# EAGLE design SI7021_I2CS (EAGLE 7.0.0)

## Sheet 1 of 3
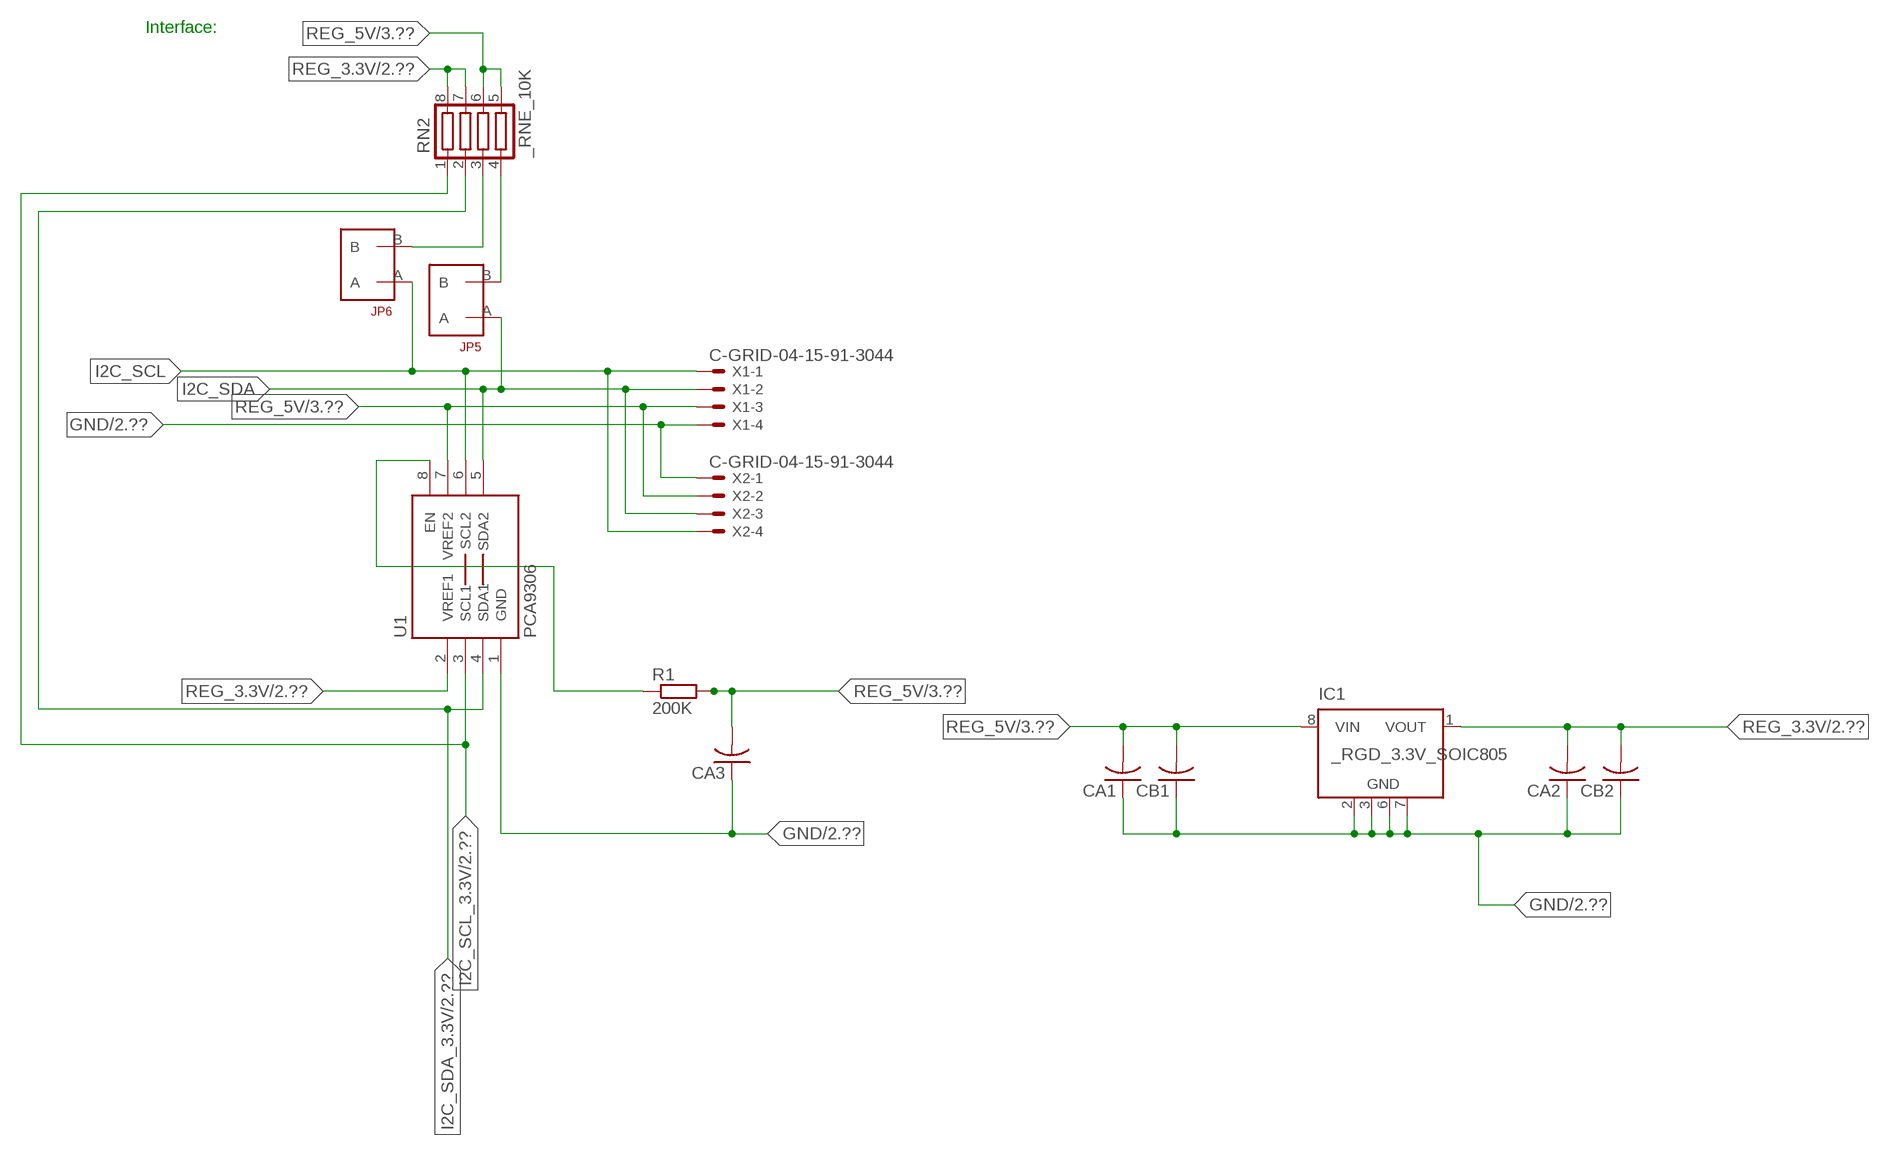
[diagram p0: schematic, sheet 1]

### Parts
CA1  CC1206KRX7R9BB104  [.1UF]
CA2  CC1206KRX7R9BB104  [.1UF]
CA3  CC1206KRX7R9BB104  [.1UF]
CB1  TMK316F106ZL-TC1206K  [TMK316F106ZL-T]
CB2  TMK316F106ZL-TC1206K  [TMK316F106ZL-T]
IC1  _RGD_3.3V_SOIC805  [_RGC_3.3V_SOIC8]
JP5  JUMPER_1X2_2MM  [JUMPER_1X2_2MM]
JP6  JUMPER_1X2_2MM  [JUMPER_1X2_2MM]
R1  200K  RESISTOR_SMT-0603  [R603]
RN2  _RNE_10K  [RNE]
U1  PCA9306  PCA9306_NCD  [PSOP-8]
X1  C-GRID-04-15-91-3044  [15-91-04]
X2  C-GRID-04-15-91-3044  [15-91-04]

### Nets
GND: CA1.1 CA2.1 CA3.1 CB1.1 CB2.1 IC1.2(GND) IC1.3(GND) IC1.6(GND) IC1.7(GND) U1.1(GND) X1.4 X2.1 ; also sheet 2,3
I2C_SCL: JP6.A U1.6(SCL2) X1.1 X2.4
I2C_SCL_3.3V: RN2.1 U1.3(SCL1) ; also sheet 2
I2C_SDA: JP5.A U1.5(SDA2) X1.2 X2.3
I2C_SDA_3.3V: RN2.2 U1.4(SDA1) ; also sheet 2
N$1: JP6.B RN2.3
N$2: JP5.B RN2.4
N$3: R1.1 U1.8(EN)
REG_3.3V: CA2.2 CB2.2 IC1.1(VOUT) RN2.7 RN2.8 U1.2(VREF1) ; also sheet 2
REG_5V: CA1.2 CA3.2 CB1.2 IC1.8(VIN) R1.2 RN2.5 RN2.6 U1.7(VREF2) X1.3 X2.2 ; also sheet 3
Unconnected: IC1.4(NC) IC1.5(NC)

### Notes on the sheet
- Interface:

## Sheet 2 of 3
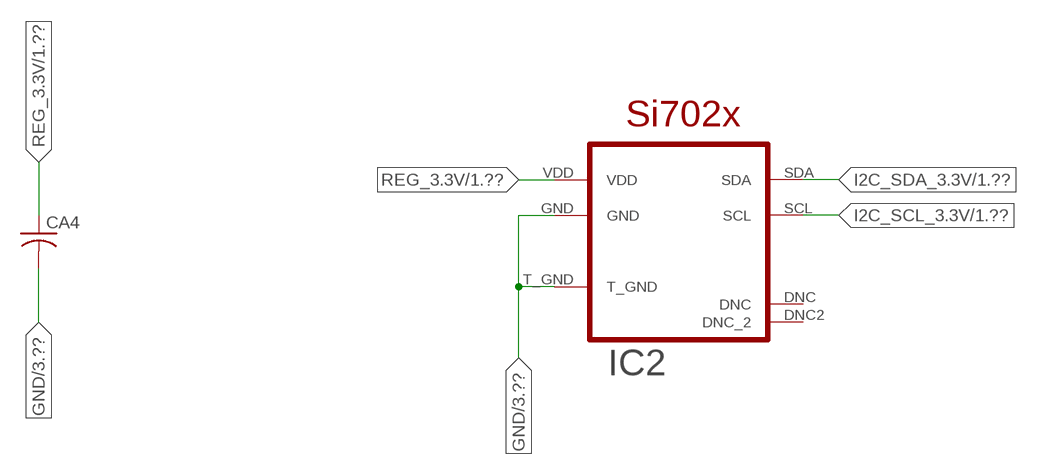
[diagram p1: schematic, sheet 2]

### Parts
CA4  CC1206KRX7R9BB104  [.1UF]
IC2  SI7021  SI702X  [DFN6]

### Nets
GND: CA4.2 IC2.GND IC2.T_GND ; also sheet 1,3
I2C_SCL_3.3V: IC2.SCL ; also sheet 1
I2C_SDA_3.3V: IC2.SDA ; also sheet 1
REG_3.3V: CA4.1 IC2.VDD ; also sheet 1
Unconnected: IC2.DNC IC2.DNC2(DNC_2)

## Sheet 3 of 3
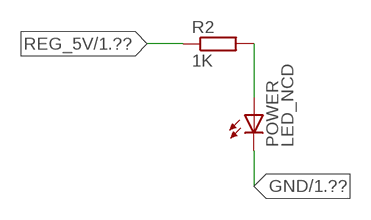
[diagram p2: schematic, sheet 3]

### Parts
POWER  LED_NCD  [CHIPLED_0603]
R2  1K  RESISTOR_SMT-0402  [R402]

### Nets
GND: POWER.C ; also sheet 1,2
N$4: POWER.A R2.2
REG_5V: R2.1 ; also sheet 1

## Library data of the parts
CA1-CA3 = NCD_ULTIMATE_LIBRARY:CC1206KRX7R9BB104: Capacitor CA .1uF 50V SMT C1206K CC1206KRX7R9BB104
CA4 = NCD_ULTIMATE_LIBRARY (1):CC1206KRX7R9BB104: Capacitor CA .1uF 50V SMT C1206K CC1206KRX7R9BB104
CB1 CB2 = NCD_ULTIMATE_LIBRARY:TMK316F106ZL-T: Capacitor CB 10uF SMT 1206 TMK316F106ZL-T
IC1 = NCD_ULTIMATE_LIBRARY:_RGD_3.3V_SOIC8: Regulator Linear 3.3V Chip Positive VOLTAGE REGULATOR Digikey 497-1199-2-ND/L78L33ACD13TR
IC2 = postalecki:SI702X
JP5 JP6 = NCD_ULTIMATE_CONNECTORS:JUMPER_1X2_2MM
POWER = NCD_ULTIMATE_LIBRARY:LED_NCD: LED Digikey 754-1132-2-ND/APT2012SRCPRV
R1 R2 = NCD_ULTIMATE_LIBRARY:RESISTOR_SMT: NCD Resistor
RN2 = NCD_ULTIMATE_LIBRARY:_RNE_10K: Resistor Array RNE SMT 10K x 4 Single Resistor Source: http://www.ctscorp.com/components/Datasheets/CTSChipArrayDs.pdf Digikey 742C083103JPTR-ND/742C083103JP; OC_FARNELL: unknown; OC_NEWARK: unknown
U1 = NCD_ULTIMATE_LIBRARY:PCA9306_NCD: NCD Bidirectional I2C level shifter. NOT compatible with all available part number pinout schemes- DOUBLE CHECK!!!; PROD_ID: IC-10023
X1 X2 = NCD_ULTIMATE_CONNECTORS:C-GRID-04: CONNECTOR 4-Pos I2C wire to board 2.54 mm (0.100") pitch header Digikey WM1342-ND/0015912045; OC_FARNELL: unknown; OC_NEWARK: unknown

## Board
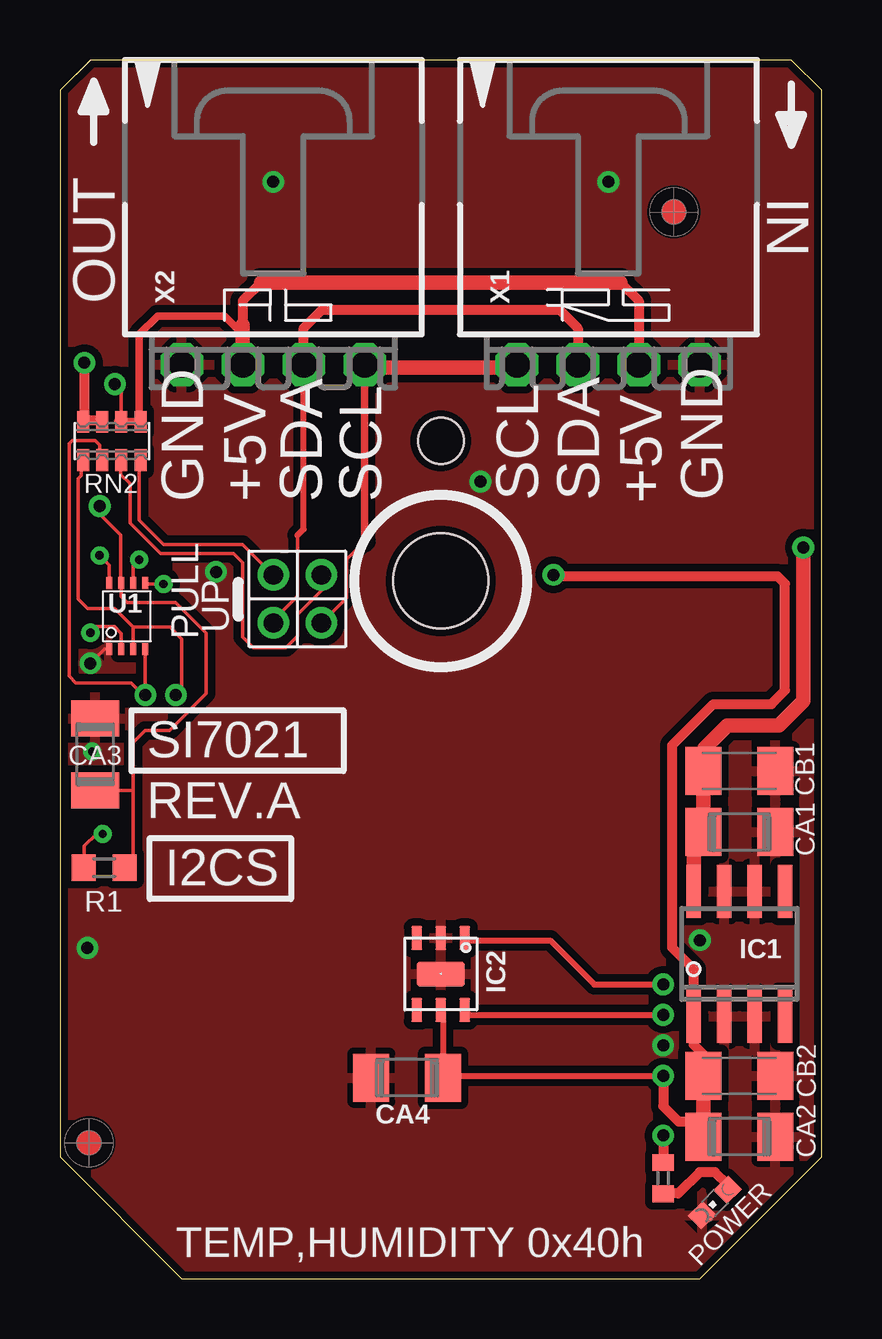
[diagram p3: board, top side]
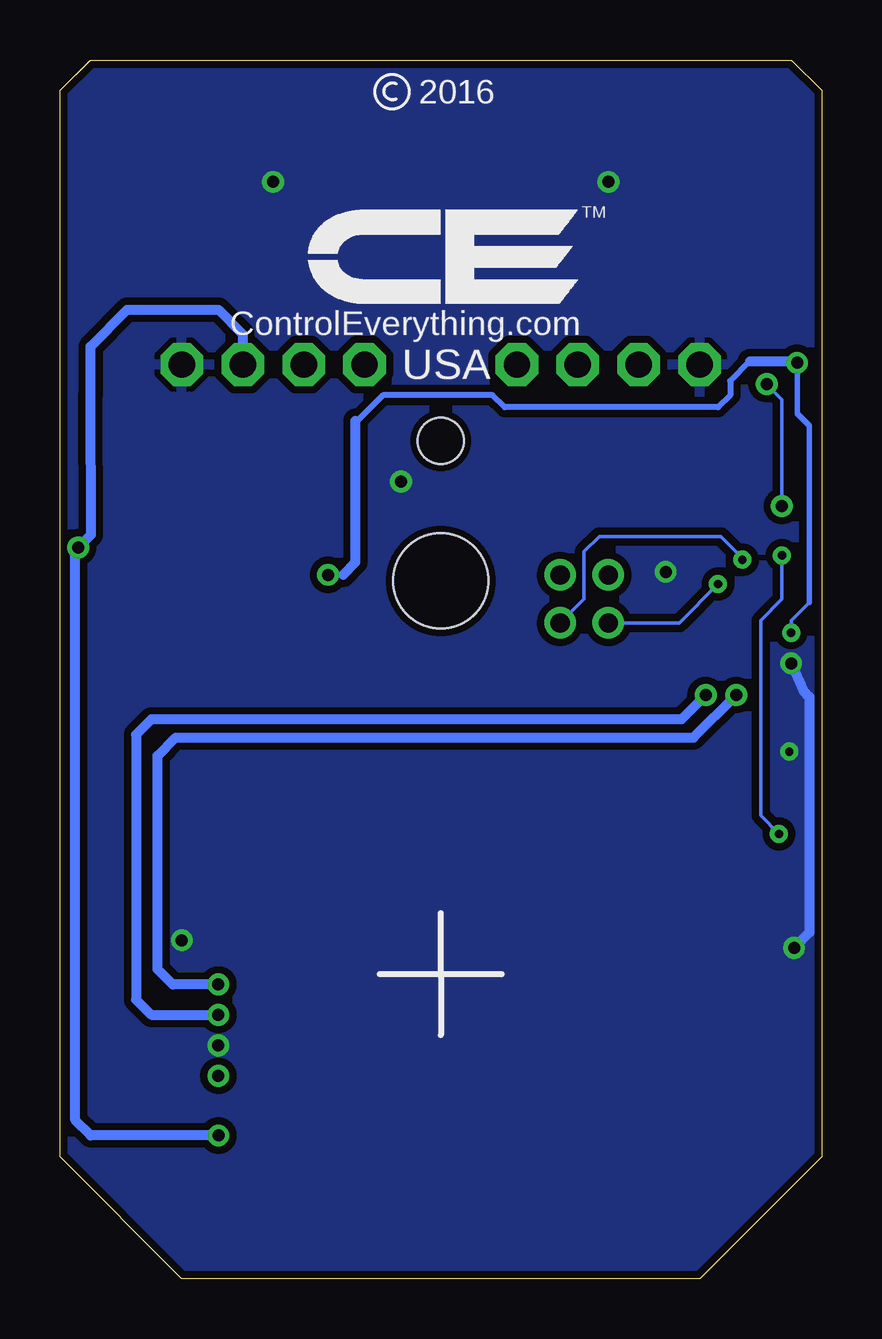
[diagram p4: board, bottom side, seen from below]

Size 31.75 x 50.8 mm. Coordinates in mm from the lower left corner, seen from the top.
Outline: 32 segments
Copper layers (1*16): Top 0.035mm / dielectric 1.5mm / Bottom 0.035mm
Design rules "default": minimum track width 5mil, minimum drill 24mil, track to track 5mil, track to pad 5mil, pad to pad 5mil, via to via 5mil, smd to smd 5mil, copper to edge 10mil, drill to drill 8mil, minimum pad ring 10mil, minimum via ring 8mil, stop-mask expansion 2mil, vias tented up to drill 0mil, thermal gap 10mil
Holes 3.96 mm at 15.88,29.08
Holes 1.91 mm at 15.88,34.93

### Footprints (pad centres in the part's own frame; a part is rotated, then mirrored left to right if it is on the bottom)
.1UF = smd 1.5 x 2: 1 -1.5,0; 2 1.5,0
TMK316F106ZL-T = smd 1.5 x 2: 1 -1.5,0; 2 1.5,0
_RGC_3.3V_SOIC8 = smd 0.6 x 2.2: 1 -1.905,-2.6; 2 -0.635,-2.6; 3 0.635,-2.6; 4 1.905,-2.6; 5 1.905,2.6; 6 0.635,2.6; 7 -0.635,2.6; 8 -1.905,2.6
DFN6 = smd 1 x 0.45: DNC -1.5,-1; DNC2 1.5,-1; GND -1.5,0; SCL 1.5,1; SDA -1.5,1; VDD 1.5,0 | smd 1 x 2: T_GND 0,0
JUMPER_1X2_2MM = drill 0.8: A 0,2; B 0,0
CHIPLED_0603 = smd 0.8 x 0.876: A 0,-0.75; C 0,0.75
R603 = smd 1 x 1.1: 1 -0.85,0; 2 0.85,0
R402 = smd 0.7 x 0.9: 1 -0.65,0; 2 0.65,0
RNE = smd 0.5 x 0.9: 1 -1.2,-0.8; 2 -0.4,-0.8; 3 0.4,-0.8; 4 1.2,-0.8; 5 1.2,0.8; 6 0.4,0.8; 7 -0.4,0.8; 8 -1.2,0.8
PSOP-8 = smd 0.25 x 0.5: 1 -0.73,-1.37; 2 -0.23,-1.37; 3 0.27,-1.37; 4 0.77,-1.37; 5 0.77,1.38; 6 0.27,1.38; 7 -0.23,1.38; 8 -0.73,1.38
15-91-04 = drill 1.1 pad 1.778 octagon: 1 -3.81,-7.62; 2 -1.27,-7.62; 3 1.27,-7.62; 4 3.81,-7.62

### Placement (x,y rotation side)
CA1  28.32,18.62 180 top
CA2  28.32,5.92 180 top
CA3  1.46,21.86 270 top
CA4  14.48,8.38 180 top
CB1  28.32,21.16 180 top
CB2  28.32,8.46 180 top
IC1  28.32,13.54 0 top
IC2  15.88,12.7 270 top
JP5  8.89,29.34 180 top
JP6  10.9,29.34 180 top
POWER  27.3,3.18 135 top
R1  1.84,17.13 0 top
R2  25.15,4.19 270 top
RN2  2.16,34.93 0 top
U1  2.79,27.61 0 top
U$5  [VISION_REF10]  1.21,5.66 90 top
U$28  [VISION_REF10]  25.59,44.46 90 top
X1  22.86,45.72 0 top
X2  8.89,45.72 0 top

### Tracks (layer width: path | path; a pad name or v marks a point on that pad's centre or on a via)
GND  (via drill 0.35, 0.5)
  Top 0.152: CA3.1 1.52,23.42 1.52,23.62 | v1.27,25.65 1.86,26.24 U1.1
  Bottom 0.406: v1.27,25.65 0.76,24.51 0.51,24.26 0.51,14.43 v1.15,13.79
  other vias: 8.89,45.72 22.86,45.72 25.15,9.73 17.53,33.22 26.67,14.11 6.5,29.46 1.35,21.97
  pour Bottom (isolate 0.305): -0.64,5.08 -0.64,49.53 1.27,51.44 30.48,51.44 32.38,49.53 32.38,5.08 26.67,-0.63 5.08,-0.63
  pour Top (isolate 0.305): 4.45,-1.27 -1.27,4.45 -1.27,50.17 0.64,52.07 31.11,52.07 33.02,50.17 33.02,4.45 27.3,-1.27
I2C_SCL  (via drill 0.35)
  Top 0.152: 12.7,30.73 11.94,29.97 11.94,28.38 JP6.A | v3.3,29.97 3.06,29.73 U1.6
  Top 0.305: 12.7,30.73 X2.4
  Top 0.406: X2.4 12.7,37.97 | 19.05,37.97 X1.1
  Top 0.61: 12.7,37.97 19.05,37.97
  Bottom 0.152: JP6.A 9.91,28.33 9.91,30.3 9.27,30.94 4.19,30.94 3.3,30.05 v3.3,29.97
I2C_SCL_3.3V  (via drill 0.5)
  Top 0.152: RN2.1 0.89,34.07 0.89,33.48 0.77,33.35 0.77,28.33 1.16,27.94 2.29,27.94 3.06,27.17 | 3.06,27.17 U1.3 | v4.83,24.33 5.08,24.59 5.08,26.67 4.58,27.17 3.06,27.17
  Top 0.254: IC2.SCL 17.08,11 v25.15,11
  Bottom 0.406: v4.83,24.33 5.84,23.32 27.94,23.32 28.58,22.68 28.58,11.63 27.94,11 v25.15,11
I2C_SDA  (via drill 0.35)
  Top 0.152: JP5.A 8.89,27.44 9.91,28.45 9.91,30.99 | U1.5 3.6,28.96 v4.32,28.96
  Top 0.254: 9.91,30.99 10.16,31.25 X2.3
  Top 0.406: 10.16,38.74 10.16,39.62 10.92,40.39 20.83,40.39 21.59,39.62 X1.2
  Top 0.61: X2.3 10.16,38.74
  Bottom 0.152: v4.32,28.96 5.94,27.34 JP5.A
I2C_SDA_3.3V  (via drill 0.5)
  Top 0.152: RN2.2 1.65,34.14 1.65,34.75 1.46,34.94 0.51,34.94 0.38,34.81 0.38,26.37 0.38,26.36 0.38,25.12 0.66,24.84 2.97,24.84 3.48,24.33 v3.56,24.33 v3.56,24.34 U1.4
  Top 0.254: IC2.SDA 16.98,14.1 20.45,14.1 22.28,12.27 v25.15,12.27
  Bottom 0.406: v25.15,12.27 27.05,12.27 27.69,12.9 27.69,21.79 26.93,22.56 5.34,22.56 v3.56,24.33
N$1
  Top 0.152: JP6.B 10.92,29.31 10.92,28.7 9.91,27.69 9.91,26.8 9.42,26.31 8.06,26.31 7.62,26.75 7.62,29.84 7.24,30.23 4.19,30.23 2.92,31.5 2.92,33.15 2.54,33.53 2.54,34.1 RN2.3
  Top 0.305: 2.54,34.02 RN2.3
N$2
  Top 0.152: JP5.B 7.62,30.61 4.32,30.61 3.3,31.62 3.3,34.07 RN2.4
  Top 0.305: 3.37,33.88 RN2.4
N$3  (via drill 0.35)
  Top 0.152: R1.1 1.02,17.16 1.02,18.03 1.52,18.54 v1.78,18.54 | v1.65,30.15 2.06,29.74 U1.8
  Bottom 0.152: v1.78,18.54 2.54,19.3 2.54,27.43 1.65,28.32 v1.65,30.15
N$4
  Top 0.406: POWER.A 27.84,3.92 27.3,4.45 26.67,4.45 25.78,3.56 25.16,3.56 R2.2
REG_3.3V  (via drill 0.35, 0.5)
  Top 0.152: v1.27,26.92 1.52,27.18 2.29,27.18 2.56,26.9 U1.2
  Top 0.254: IC2.VDD 15.98,11.1 CA4.1 16.05,8.46 v25.15,8.46
  Top 0.406: CB2.2 26.82,9.35 26.42,9.75 26.42,10.36 | v25.15,8.46 25.15,7.19 25.78,6.55 26.82,6.55 | IC1.1 26.42,12.9 25.53,13.79 25.53,22.24 27.24,23.95 29.66,23.95 30.23,24.52 30.23,28.97 29.91,29.29 20.62,29.29 v20.57,29.34 | 26.52,5.62 CA2.2 | v1.02,38.18 1.02,35.78 | 1.02,35.78 RN2.8 | 1.02,35.78 1.71,35.78 RN2.7
  Top 0.61: CB2.2 26.82,6.55 CA2.2 | 26.42,10.36 IC1.1
  Bottom 0.152: 0.51,28.19 1.27,27.43 v1.27,26.92
  Bottom 0.229: 0.51,28.19 0.51,35.56 1.02,36.07 v1.02,38.18
  Bottom 0.254: 19.94,29.34 v20.57,29.34 | 2.99,38.24 3.81,37.42 3.81,36.83 4.32,36.32 13.21,36.32 13.72,36.83 18.29,36.83 19.36,35.76 19.43,35.76
  Bottom 0.406: 19.94,29.34 19.43,29.87 19.43,35.76 | 2.99,38.24 1.08,38.24 v1.02,38.18
REG_5V  (via drill 0.5)
  Top 0.152: RN2.6 2.56,37.01 v2.29,37.29 | R1.2 3.05,17.49 3.05,20.36 | 3.05,20.36 3.05,22.35 3.56,22.86 4.57,22.86 6.1,24.38 6.1,26.92 4.83,28.19 2.79,28.19 2.56,28.43 U1.7 2.54,29.01 2.54,30.99 1.65,31.87 v1.65,32.21 | CA3.2 3.05,20.36
  Top 0.305: 7.5,39.37 7.62,39.37 6.86,40.13 4.07,40.13 3.31,39.37 3.31,35.8 RN2.5 RN2.6 2.42,35.74
  Top 0.406: v25.15,5.97 R2.1 | 8.38,41.53 7.62,40.77 7.62,39.37 | 23.37,41.53 24.13,40.77 X1.3
  Top 0.61: X2.2 7.62,39.37 7.62,39.75 | 8.38,41.53 23.37,41.53 | IC1.8 26.42,18.21 CA1.2 CB1.2 26.86,21.2 26.86,22.11 27.82,23.06 29.98,23.06 30.99,24.08 v30.99,30.48
  Bottom 0.152: v1.65,32.21 1.65,36.65 v2.29,37.29
  Bottom 0.406: v25.15,5.97 30.48,5.97 31.11,6.6 31.11,30.36 v30.99,30.48 30.47,31 30.48,36.83 30.48,38.86 28.96,40.39 25.15,40.39 24.13,39.37 X1.3

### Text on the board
tNames: IN | OUT | GND | +5V | SDA | SCL | SCL | SDA | +5V | GND | PULL | UP | SI7021 | REV.A | I2CS | TEMP,HUMIDITY 0x40h
bNames: 2016 | TM | ControlEverything.com | USA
